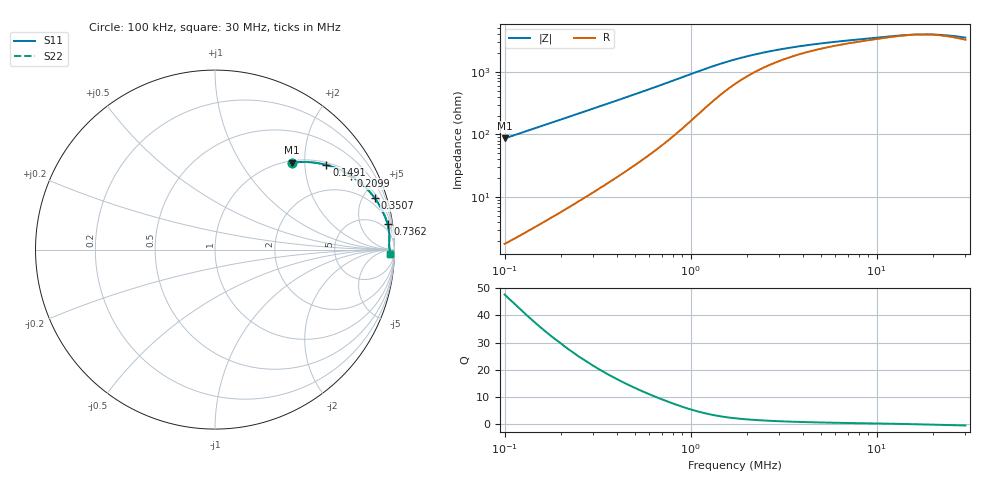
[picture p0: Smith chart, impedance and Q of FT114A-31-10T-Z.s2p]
! ListType=Log
!!FT114A-31 10T Z
# MHZ S RI R 50
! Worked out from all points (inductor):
!   101 points, 100 kHz to 30 MHz, reference 50 ohm
!   read as one part in series: L = 137 uH near 100 kHz
!   highest Q = 47.7 at 100 kHz (marker M1), where L = 138 uH
!   self-resonance near 17.08 MHz
!   S11 on the Smith chart (normalised r, x): 100 kHz: 1.04, +1.73; 149.1 kHz: 1.07, +2.57; 209.9 kHz: 1.13, +3.62; 350.7 kHz: 1.33, +6.06; 736.2 kHz: 3, +13; 30 MHz: 39, -37
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0.1  0.4298 0.4844  0.5704 -0.4848  0.571 -0.4847  0.4293 0.4843
0.1186625  0.5126 0.488  0.4875 -0.4885  0.4881 -0.4885  0.5121 0.488
0.1490728  0.6206 0.4715  0.3795 -0.472  0.38 -0.4721  0.6201 0.4716
0.1768936  0.6944 0.4452  0.3056 -0.4457  0.306 -0.4459  0.694 0.4454
0.2099064  0.7589 0.4103  0.2412 -0.4109  0.2416 -0.4111  0.7584 0.4105
0.2637003  0.8281 0.3566  0.1718 -0.357  0.1721 -0.3573  0.8278 0.3568
0.350725  0.8896 0.2874  0.1103 -0.2878  0.1105 -0.2881  0.8893 0.2876
0.4938487  0.9345 0.2126  0.0653 -0.2131  0.0654 -0.2133  0.9344 0.2128
0.6953784  0.9586 0.1517  0.0412 -0.1522  0.0413 -0.1524  0.9584 0.1519
0.7361943  0.9612 0.1429  0.0386 -0.1435  0.0387 -0.1436  0.961 0.143
1.302281  0.9716 0.0752  0.0281 -0.0759  0.0281 -0.0761  0.9716 0.0753
1.833715  0.9711 0.051  0.0286 -0.0521  0.0287 -0.0522  0.9711 0.0511
2.175933  0.9706 0.0423  0.0291 -0.0436  0.0291 -0.0437  0.9706 0.0424
2.733571  0.9704 0.0331  0.0293 -0.0347  0.0293 -0.0347  0.9704 0.0332
3.434118  0.9704 0.0258  0.0293 -0.0277  0.0293 -0.0278  0.9704 0.0259
4.567423  0.9707 0.0185  0.029 -0.021  0.029 -0.021  0.9707 0.0185
6.431296  0.9714 0.0114  0.0282 -0.0148  0.0282 -0.0148  0.9714 0.0114
12.04431  0.9736 -0.000534  0.026 -0.00577  0.026 -0.00579  0.9736 -0.000465
16.01909  0.9745 -0.007  0.0251 -0.00128  0.0251 -0.0013  0.9745 -0.00699
20.12439  0.9745 -0.013  0.0249 0.00257  0.0249 0.00254  0.9745 -0.013
25.28178  0.9739 -0.0197  0.0254 0.00668  0.0254 0.00665  0.974 -0.0196
30  0.9732 -0.0249  0.0262 0.0099  0.0262 0.00987  0.9732 -0.025
